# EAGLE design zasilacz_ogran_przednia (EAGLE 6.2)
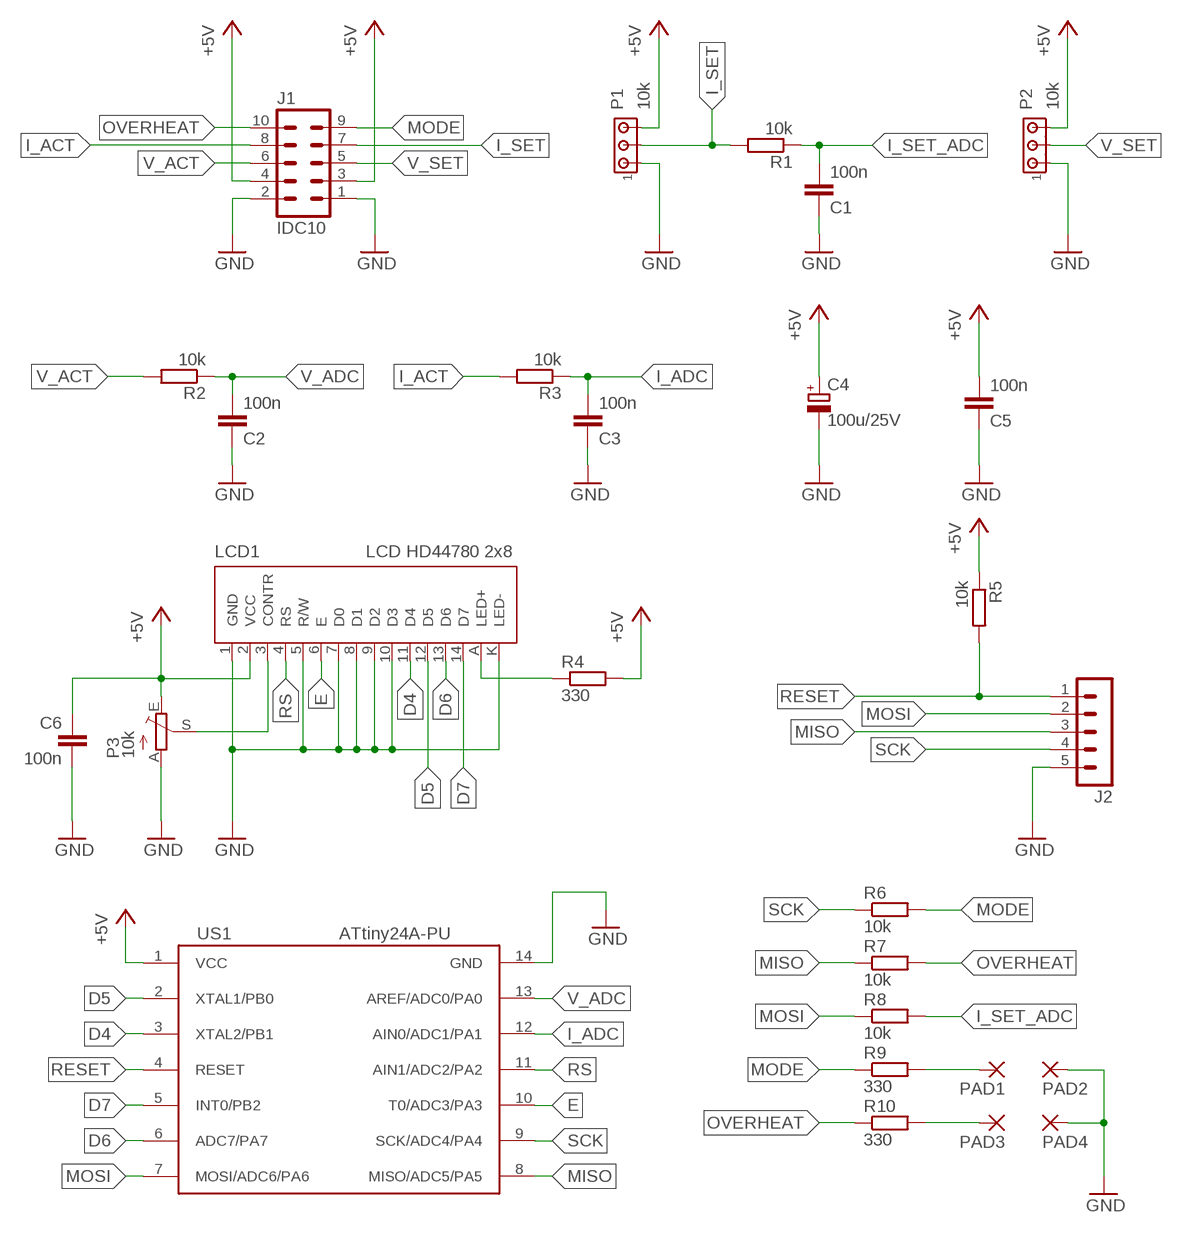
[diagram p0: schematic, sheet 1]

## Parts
C1  100n  C-EU050-025X075  [C050-025X075]
C2  100n  C-EU050-025X075  [C050-025X075]
C3  100n  C-EU050-025X075  [C050-025X075]
C4  100u/25V  CPOL-EUE2.5-6  [E2,5-6]
C5  100n  C-EU050-025X075  [C050-025X075]
C6  100n  C-EU050-025X075  [C050-025X075]
J1  IDC10  ML10  [ML10]
J2  MA05-1  [MA05-1]
LCD1  LCD HD44780 2x8  LCD_ZLACZE-MINI  [LCD_HD44780_1X6_NAD-ELEMENTAMI_Z-PODSW]
P1  10k  ARK3-5MM  [3PIN-5MM]
P2  10k  ARK3-5MM  [3PIN-5MM]
P3  10k  TRIM_EU-CA6V  [CA6V]
PAD1  SMD5  [SMD2,54-5,08]
PAD2  SMD5  [SMD2,54-5,08]
PAD3  SMD5  [SMD2,54-5,08]
PAD4  SMD5  [SMD2,54-5,08]
R1  10k  R-EU_0207/7  [0207/7]
R2  10k  R-EU_0207/7  [0207/7]
R3  10k  R-EU_0207/7  [0207/7]
R4  330  R-EU_0207/7  [0207/7]
R5  10k  R-EU_0207/7  [0207/7]
R6  10k  R-EU_0207/7  [0207/7]
R7  10k  R-EU_0207/7  [0207/7]
R8  10k  R-EU_0207/7  [0207/7]
R9  330  R-EU_0207/7  [0207/7]
R10  330  R-EU_0207/7  [0207/7]
US1  ATtiny24A-PU  ATTINY24/44/84-PU  [DIL14]

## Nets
+5V: C4.+ C5.2 C6.1 J1.3 J1.4 LCD1.2(VCC) P1.P$3 P2.P$3 P3.E R4.2 R5.1 US1.1(VCC)
D4: LCD1.11(D4) US1.3(XTAL2/PB1)
D5: LCD1.12(D5) US1.2(XTAL1/PB0)
D6: LCD1.13(D6) US1.6(ADC7/PA7)
D7: LCD1.14(D7) US1.5(INT0/PB2)
E: LCD1.6(E) US1.10(T0/ADC3/PA3)
GND: C1.1 C2.1 C3.1 C4.- C5.1 C6.2 J1.1 J1.2 J2.5 LCD1.1(GND) LCD1.5(R/W) LCD1.7(D0) LCD1.8(D1) LCD1.9(D2) LCD1.10(D3) LCD1.K(LED-) P1.P$1 P2.P$1 P3.A PAD2.1(P) PAD4.1(P) US1.14(GND)
I_ACT: J1.8 R3.2
I_ADC: C3.2 R3.1 US1.12(AIN0/ADC1/PA1)
I_SET: J1.7 P1.P$2 R1.2
I_SET_ADC: C1.2 R1.1 R8.2
MISO: J2.3 R7.1 US1.8(MISO/ADC5/PA5)
MODE: J1.9 R6.2 R9.1
MOSI: J2.2 R8.1 US1.7(MOSI/ADC6/PA6)
N$1: LCD1.3(CONTR) P3.S
N$2: PAD1.1(P) R9.2
N$3: PAD3.1(P) R10.2
N$5: LCD1.A(LED+) R4.1
OVERHEAT: J1.10 R7.2 R10.1
RESET: J2.1 R5.2 US1.4(RESET)
RS: LCD1.4(RS) US1.11(AIN1/ADC2/PA2)
SCK: J2.4 R6.1 US1.9(SCK/ADC4/PA4)
V_ACT: J1.6 R2.2
V_ADC: C2.2 R2.1 US1.13(AREF/ADC0/PA0)
V_SET: J1.5 P2.P$2

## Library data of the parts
C1-C3 C5 C6 = rcl:C-EU: CAPACITOR, European symbol
C4 = rcl:CPOL-EU: POLARIZED CAPACITOR, European symbol
J1 = con-ml:ML10: HARTING; OC_FARNELL: unknown; OC_NEWARK: unknown
J2 = zlacza_futrzak:MA05-1: PIN HEADER; OC_FARNELL: unknown; OC_NEWARK: unknown
LCD1 = inne_futrzak:LCD_ZLACZE
P1 P2 = zlacza_futrzak:ARK3: ARK 3 Raster 5mm i 3,5mm
P3 = pot:TRIM_EU-: POTENTIOMETER
PAD1-PAD4 = wirepad:SMD5: SMD PAD
R1-R10 = rcl:R-EU_: RESISTOR, European symbol
US1 = scalaki_futrzak:ATTINY24/44/84

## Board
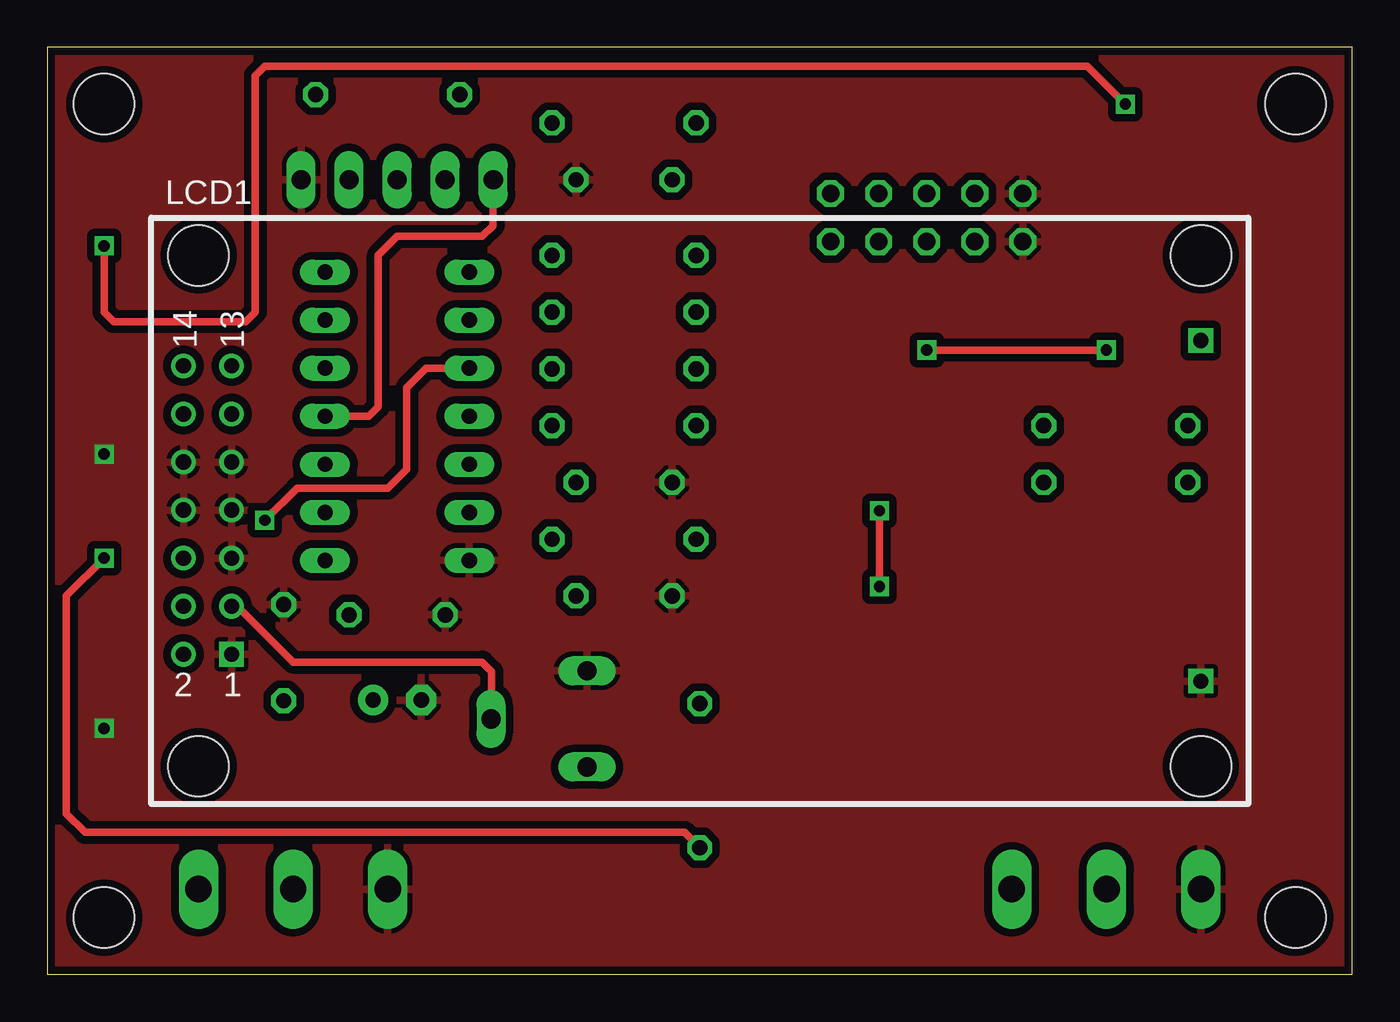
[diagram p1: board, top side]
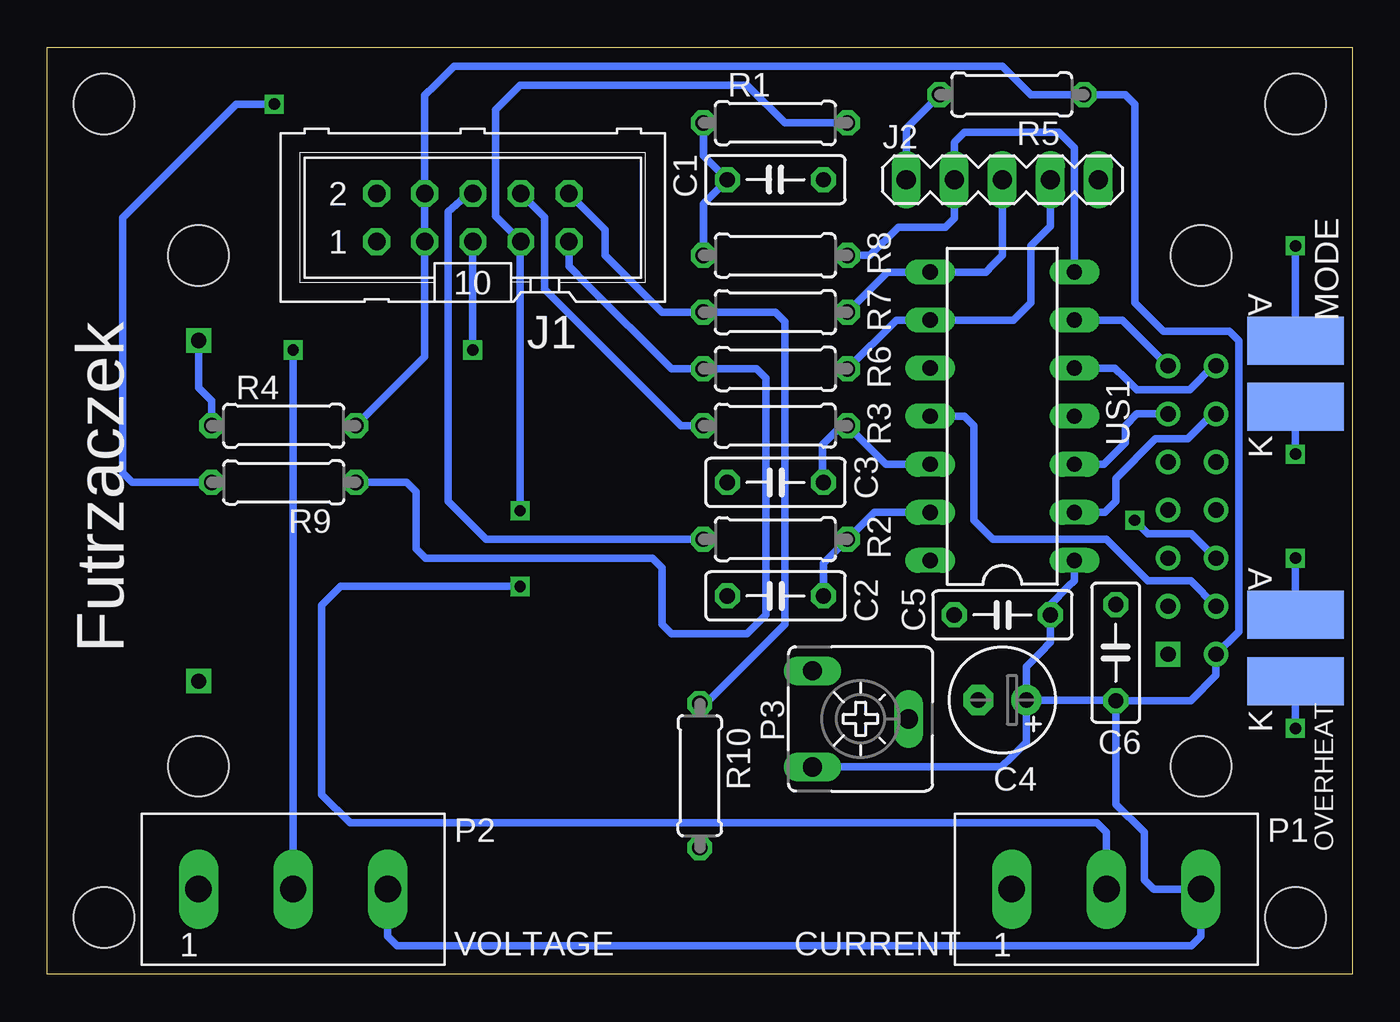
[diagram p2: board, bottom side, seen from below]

Size 69 x 49 mm. Coordinates in mm from the lower left corner, seen from the top.
Outline: 0,0 69,0 69,49 0,49 0,0
Copper layers (1*16): Top 0.035mm / dielectric 1.5mm / Bottom 0.035mm
Design rules: minimum track width 10mil, minimum drill 22mil, track to track 8mil, track to pad 8mil, pad to pad 8mil, via to via 8mil, smd to smd 8mil, copper to edge 15mil, drill to drill 8mil, minimum pad ring 10mil, minimum via ring 8mil, stop-mask expansion 4mil, vias tented up to drill 0mil, thermal gap 10mil
Holes 3.2 mm at 3,3 66,3 3,46 66,46

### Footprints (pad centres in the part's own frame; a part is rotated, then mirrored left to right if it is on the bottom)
C050-025X075 = drill 0.813 octagon: 1 -2.54,0; 2 2.54,0
E2,5-6 = drill 0.813 pad 1.6: + -1.27,0 | drill 0.813 pad 1.6 octagon: - 1.27,0
ML10 = drill 0.914 octagon: 1 -5.08,-1.27; 2 -5.08,1.27; 3 -2.54,-1.27; 4 -2.54,1.27; 5 0,-1.27; 6 0,1.27; 7 2.54,-1.27; 8 2.54,1.27; 9 5.08,-1.27; 10 5.08,1.27
MA05-1 = drill 1.016 long: 1 -5.08,0; 2 -2.54,0; 3 0,0; 4 2.54,0; 5 5.08,0
LCD_HD44780_1X6_NAD-ELEMENTAMI_Z-PODSW = drill 0.8 square: 1 1.74,5.92; A 53,22.5; K 53,4.5 | drill 0.8: 2 -0.8,5.92; 3 1.74,8.46; 4 -0.8,8.46; 5 1.74,11; 6 -0.8,11; 7 1.74,13.54; 8 -0.8,13.54; 9 1.74,16.08; 10 -0.8,16.08; 11 1.74,18.62; 12 -0.8,18.62; 13 1.74,21.16; 14 -0.8,21.16 | hole 3.2: 0,0; 0,27; 53,0; 53,27
3PIN-5MM = drill 1.4 long: P$1 -5,0; P$2 0,0; P$3 5,0
CA6V = drill 1.016 long: A -2.54,-2.54; E 2.54,-2.54; S 0,2.54
SMD2,54-5,08 = smd 2.54 x 5.08: 1 0,0
0207/7 = drill 0.813 octagon: 1 -3.81,0; 2 3.81,0
DIL14 = drill 0.813 long: 1 -7.62,-3.81; 2 -5.08,-3.81; 3 -2.54,-3.81; 4 0,-3.81; 5 2.54,-3.81; 6 5.08,-3.81; 7 7.62,-3.81; 8 7.62,3.81; 9 5.08,3.81; 10 2.54,3.81; 11 0,3.81; 12 -2.54,3.81; 13 -5.08,3.81; 14 -7.62,3.81

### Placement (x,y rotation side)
C1  30.5,42 180 bottom
C2  30.5,20 0 bottom
C3  30.5,26 0 bottom
C4  18.5,14.5 180 bottom
C5  18.5,19 0 bottom
C6  12.5,17 90 bottom
J1  46.5,40 0 bottom
J2  18.5,42 0 bottom
LCD1  8,11 0 top
P1  13,4.5 0 bottom
P2  56,4.5 0 bottom
P3  26,13.5 270 bottom
PAD1  3,33.5 270 bottom
PAD2  3,30 270 bottom
PAD3  3,19 270 bottom
PAD4  3,15.5 270 bottom
R1  30.5,45 0 bottom
R2  30.5,23 180 bottom
R3  30.5,29 180 bottom
R4  56.5,29 0 bottom
R5  18,46.5 180 bottom
R6  30.5,32 180 bottom
R7  30.5,35 180 bottom
R8  30.5,38 180 bottom
R9  56.5,26 180 bottom
R10  34.5,10.5 270 bottom
US1  18.5,29.5 90 bottom

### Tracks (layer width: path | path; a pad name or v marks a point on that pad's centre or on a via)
+5V
  Bottom 0.406: US1.1 14.69,20.81 15,20.5 15.96,19.54 C5.2 15.96,17.54 16.5,17 17.23,16.27 C4.+ | C6.1 8.54,14.46 8.5,14.5 7.2,15.8 LCD1.2 6,18.12 6,33.5 6.5,34 10,34 11.5,35.5 11.5,46 12,46.5 R5.1 17,46.5 18.5,48 47.5,48 48.5,47 49.04,46.46 J1.4 J1.3 49.04,32.65 R4.2 | C4.+ 12.54,14.5 C6.1 | P2.P$3 51,2 50.5,1.5 8.5,1.5 8,2 P1.P$3 10.5,4.5 11,5 11,7.5 12.5,9 C6.1 | C4.+ 17.23,12.27 18,11.5 18.54,10.96 P3.E
D4
  Bottom 0.406: LCD1.11 10.38,29.62 11.38,29.62 12,29 12,28.1 13.14,26.96 US1.3
D5
  Bottom 0.406: LCD1.12 7.38,29.62 8.7,28.3 10.4,28.3 12.5,26.2 12.5,25 13.08,24.42 US1.2
D6
  Bottom 0.406: US1.6 12.16,34.58 LCD1.13
D7
  Bottom 0.406: LCD1.14 7.34,32.16 8.6,30.9 11.4,30.9 12,31.5 12.54,32.04 US1.5
E  (via drill 0.6)
  Top 0.406: US1.10 20.04,32.04 19,31 19,26.7 18,25.7 13.2,25.7 v11.5,24
  Bottom 0.406: v11.5,24 10.8,23.3 8.5,23.3 LCD1.6
GND  (via drill 0.6)
  Bottom 0.406: PAD4.1 v3,13 | PAD2.1 v3,27.5
  pour Top (isolate 0.406): 0,0 69,0 69,49 0,49
I_ACT
  Bottom 0.406: R3.2 35.5,29 42.7,36.2 42.7,40.01 J1.8
I_ADC
  Bottom 0.406: C3.2 28,26.04 28,28 27,29 R3.1 24.65,26.96 US1.12
I_SET  (via drill 0.6)
  Top 0.406: v44,20.5 v44,24.5
  Bottom 0.406: R1.2 30,45 32,47 44,47 45.3,45.7 45.3,45.5 45.3,40.07 J1.7 44,38.69 v44,24.5 | P1.P$2 13,7.5 13.5,8 41.5,8 53,8 54.5,9.5 54.5,19.5 53.5,20.5 v44,20.5
I_SET_ADC
  Bottom 0.406: R1.1 34.31,43.27 C1.2 34.31,40.73 R8.2
MISO
  Bottom 0.406: J2.3 18.5,38 19,37.5 19.38,37.12 US1.8 24.57,37.12 R7.1
MODE
  Bottom 0.406: J1.9 41.42,37.42 40.5,36.5 36,32 R6.2 31.5,32 31,31.5 31,19 32,18 36,18 36.5,18.5 36.5,21.5 37,22 49,22 49.5,22.5 49.5,25.5 50,26 R9.1
MOSI
  Bottom 0.406: US1.7 14.69,43.69 15.5,44.5 20.5,44.5 21,44 21.04,43.96 J2.2 21.04,39.96 21.5,39.5 24,39.5 25.5,38 R8.1
N$1
  Top 0.406: LCD1.3 10.04,19.46 13,16.5 23,16.5 23.5,16 23.5,13.54 P3.S
N$2  (via drill 0.6)
  Top 0.406: v57,46 55,48 11.5,48 11,47.5 11,35 10.5,34.5 3.5,34.5 3,35 v3,38.5
  Bottom 0.406: R9.2 64.5,26 65,26.5 65,40 59,46 v57,46 | v3,38.5 PAD1.1
N$3  (via drill 0.6)
  Top 0.406: v3,22 1,20 1,8.5 2,7.5 30,7.5 33.69,7.5 R10.2
  Bottom 0.406: PAD3.1 v3,22
N$5
  Bottom 0.406: LCD1.A 61,31 60.5,30.5 60.31,30.31 R4.1
OVERHEAT
  Bottom 0.406: J1.10 39.5,39.35 39.5,38 36.5,35 R7.2 30.5,35 30,34.5 30,18.5 32.5,16 33.5,15 34.19,14.31 R10.1
RESET
  Top 0.406: US1.4 17,29.5 17.5,30 17.5,38 18.5,39 23,39 23.58,39.58 J2.1
  Bottom 0.406: J2.1 23.58,44.73 R5.2
RS
  Bottom 0.406: US1.11 20.5,29.5 20,29 20,24 19,23 13,23 12.5,22.5 10.8,20.8 8.54,20.8 LCD1.4
SCK
  Bottom 0.406: J2.4 15.96,39.54 17,38.5 17,35.5 17.5,35 17.92,34.58 US1.9 24.11,34.58 R6.1
V_ACT
  Bottom 0.406: J1.6 46.73,41.27 47.8,40.3 47.8,25 45.8,23 R2.2
V_ADC
  Bottom 0.406: US1.13 25.27,24.42 R2.1 27.96,21.73 C2.2
V_SET  (via drill 0.6)
  Top 0.406: v56,33 v46.5,33
  Bottom 0.406: P2.P$2 v56,33 | v46.5,33 J1.5

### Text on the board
bPlace: MODE | A | Futrzaczek | K | A | K | OVERHEAT | CURRENT | VOLTAGE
